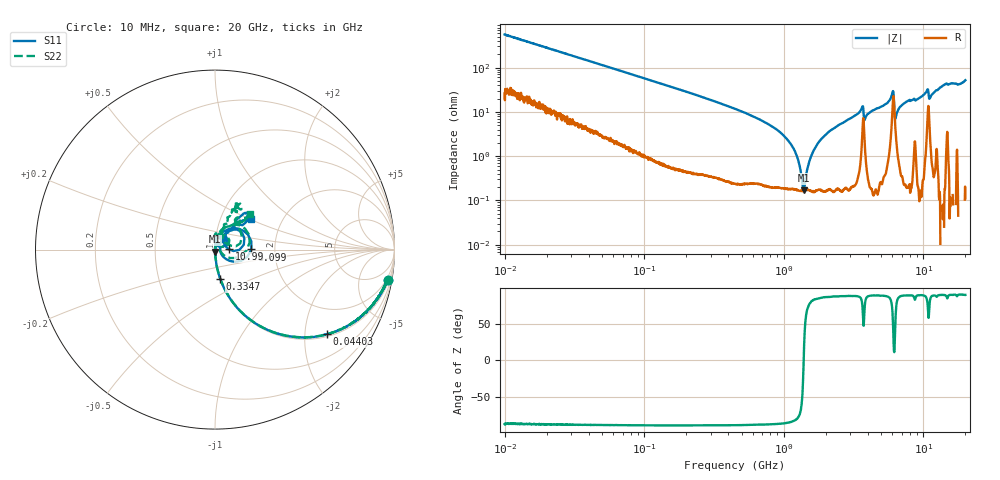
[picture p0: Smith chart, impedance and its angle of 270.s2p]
!Keysight Technologies,P5008B,MY61100088,A.16.20.02
!Date: Friday, August 30, 2024 13:53:25
!Correction: S11(C  2-Port  )
!S21(C  2-Port  )
!S12(C  2-Port  )
!S22(C  2-Port  )
!S2P File: Measurements: S11, S21, S12, S22:Log Frequency Sweep
# Hz S  MA  R 50
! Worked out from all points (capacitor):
!   1601 points, 10 MHz to 20 GHz, reference 50 ohm
!   read as one part in series: C = 28.4 pF near 10.39 MHz
!   lowest |Z| = 171 mohm at 1.385 GHz (marker M1)
!   series resonance near 1.388 GHz, so ESL is about 460 pH
!   S11 on the Smith chart (normalised r, x): 10 MHz: 1, -11; 44.03 MHz: 1.07, -2.58; 334.7 MHz: 1.00, -0.34; 6.099 GHz: 1.51, +0.00; 10.99 GHz: 1.17, +0.00; 20 GHz: 1.39, +0.51
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1e7  0.9771 -10.0  0.1743 77.3  0.1743 77.3  0.9765 -10.0
3.555162e7  0.8368 -31.6  0.5229 56.7  0.5228 56.7  0.8367 -31.5
4.402515e7  0.7805 -37.2  0.6036 51.2  0.6035 51.2  0.7804 -37.1
1.263918e8  0.4126 -65.0  0.9045 24.2  0.9043 24.2  0.4127 -64.9
3.347058e8  0.165 -79.9  0.9832 9.2  0.9831 9.1  0.1649 -79.6
4.472136e8  0.1204 -82.5  0.9903 6.5  0.99 6.4  0.1204 -82.6
9.428195e8  0.04272 -85.9  0.9971 1.5  0.9967 1.5  0.04264 -86.6
1.385298e9  0.01148 -85.0  0.9982 -0.6  0.9979 -0.6  0.01144 -81.1
1.589917e9  0.003208 -57.1  0.9984 -1.4  0.9981 -1.4  0.00308 -71.4
1.675209e9  0.001244 41.2  0.9984 -1.7  0.998 -1.7  0.002124 19.4
1.842179e9  0.008588 63.6  0.9984 -2.3  0.9981 -2.3  0.007679 89.3
2.185773e9  0.01966 79.3  0.9983 -3.3  0.9979 -3.4  0.01903 84.0
3.582383e9  0.07681 74.8  0.9869 -8.4  0.9868 -8.4  0.07682 72.4
3.902191e9  0.04214 84.5  0.9936 -6.9  0.9933 -6.9  0.04416 65.5
5.652411e9  0.1034 69.2  0.9863 -13.7  0.9861 -13.8  0.1076 71.8
6.098795e9  0.2027 0.3  0.8117 -12.1  0.8115 -12.2  0.1977 12.1
6.549245e9  0.03333 32.1  0.9915 -10.6  0.9912 -10.7  0.02598 80.5
7.697294e9  0.08314 59.0  0.9977 -15.4  0.9974 -15.5  0.08081 84.3
1.048196e10  0.1393 49.6  0.9773 -24.4  0.9769 -24.6  0.1365 65.5
1.099193e10  0.07764 0.9  0.9304 -19.0  0.9301 -19.2  0.09318 13.4
1.413906e10  0.268 49.6  0.9736 -31.5  0.9732 -31.7  0.2668 63.7
2e10  0.2642 40.6  0.9633 -46.8  0.963 -47.0  0.2779 45.3
